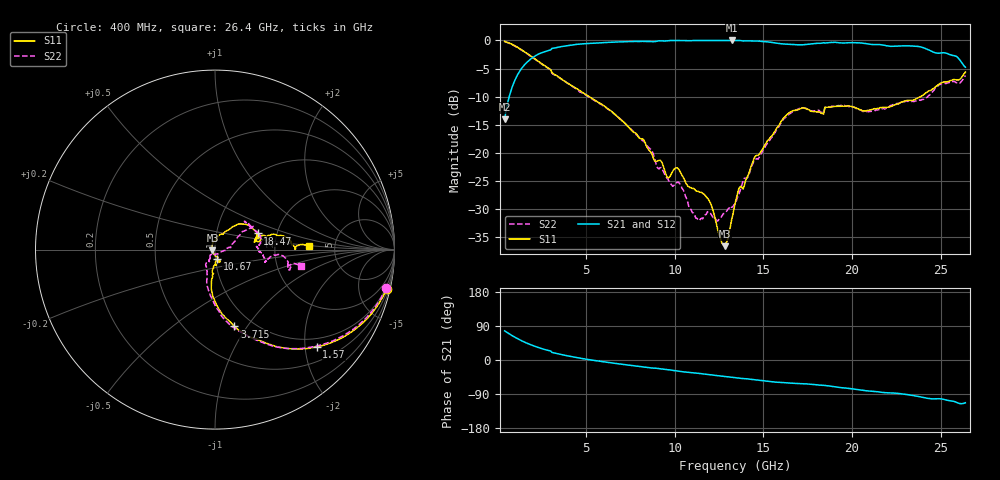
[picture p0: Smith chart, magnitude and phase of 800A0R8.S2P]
!  American Technical Ceramics  Date:  9/12/2007
!  One Norden Lane
!  Huntington Station,  NY.  11746-2102
!  Tel:  (631) 622-4700  Fax:  (631) 622-4748
!  Part Number  800A0R8  Mounting Orientation: Vertical
!  Description: Ultra Low ESR Microwave capacitors
!  Application: Coupling, Bypass, Tuning, DC Block
!  Filters, Matching
# GHZ S DB R 50
! Freq  |S11|  S11 Ph  |S21|  S21 Ph  |S12|  S12 Ph  |S22|  S22 Ph
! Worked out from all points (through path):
!   401 points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, 400 MHz to 26.4 GHz, reference 50 ohm
!   highest |S21| = 0.00 dB at 13.21 GHz (marker M1); lowest = -14.0 dB at 400 MHz (marker M2)
!   lowest |S11| = -36.6 dB at 12.81 GHz (marker M3), VSWR 1.03, Z = 48.6 - j0.368 ohm
!   |S11| at or under -10 dB: 5.18 GHz to 23.88 GHz (18.7 GHz wide, 129 % of centre)
!   |S22| runs from -32.1 to -0.2 dB; largest |S21 - S12| = 0.0079
!   S11 on the Smith chart (normalised r, x): 400 MHz: 0.72, -8.76; 1.57 GHz: 0.80, -2.25; 3.715 GHz: 0.82, -0.87; 10.67 GHz: 1.02, -0.10; 18.47 GHz: 1.59, +0.31; 26.4 GHz: 3.18, +0.16
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0.4  -0.16 -12.9  -14.05 76.9  -14.06 76.9  -0.21 -12.7
0.92  -0.85 -28.3  -7.52 61.7  -7.53 61.7  -0.89 -27.9
1.57  -2.12 -43.7  -4.17 46.2  -4.19 46.2  -2.15 -43.6
3.715  -7.10 -75.8  -1.03 13.2  -1.04 13.3  -7.08 -76.9
4.755  -9.14 -84.7  -0.62 4.0  -0.62 4.1  -9.28 -86.2
7.095  -14.43 -96.0  -0.24 -11.7  -0.23 -11.5  -14.44 -103.9
9.11  -21.32 -83.9  -0.06 -22.9  -0.04 -22.7  -22.83 -115.7
9.63  -24.44 -75.3  -0.03 -25.6  -0.01 -25.5  -24.76 -117.8
10.15  -22.66 -72.7  -0.01 -29.4  -0.01 -29.3  -25.15 -115.4
10.67  -25.57 -75.7  -0.04 -32.2  -0.02 -32.1  -28.13 -130.5
11.32  -26.82 -68.2  -0.01 -35.1  -0.01 -35.1  -31.88 -109.0
11.905  -28.28 -80.3  -0.01 -38.7  -0.01 -38.7  -30.44 -89.5
12.815  -36.57 -165.2  -0.01 -43.5  -0.01 -43.5  -30.72 -51.5
13.205  -31.95 127.8  0.00 -45.6  -0.01 -45.6  -29.66 -35.8
13.4  -29.06 112.0  0.00 -46.4  -0.01 -46.5  -29.08 -23.5
14.505  -20.77 69.9  -0.11 -52.0  -0.08 -52.1  -21.31 8.8
16.13  -13.84 44.8  -0.63 -59.7  -0.60 -59.9  -14.02 32.3
17.755  -12.61 15.1  -0.60 -64.1  -0.56 -64.3  -12.49 35.3
18.47  -11.90 20.7  -0.46 -67.2  -0.43 -67.4  -11.91 22.5
22.11  -11.82 16.0  -1.03 -86.9  -1.00 -87.2  -11.73 -3.9
23.8  -10.09 14.7  -1.10 -96.9  -1.08 -97.3  -10.58 -11.7
26.4  -5.63 2.1  -4.76 -112.9  -4.75 -113.2  -6.23 -10.7
